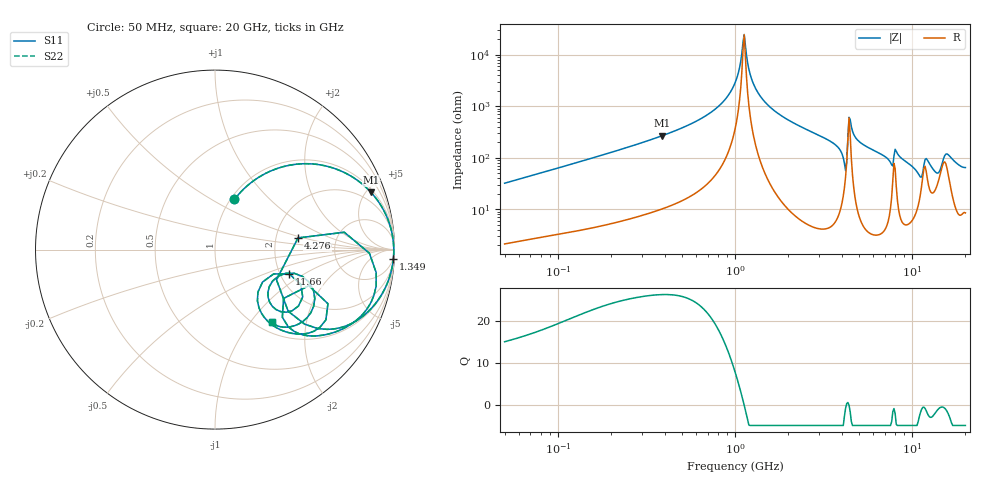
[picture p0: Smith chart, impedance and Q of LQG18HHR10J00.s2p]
!Murata Part Number: LQG18HHR10J00
!These Parameters are Measured in Series Mode Connection
!  o--[Z]--o
!Port1  Port2
!  o-------o
!Freq. Start=50[MHz] Stop=20[GHz], 401[Steps]
# Hz S RI R 50
!Freq.(Hz) S11(Real) S11(Imag) S21(Real) S21(Imag) S12(Real) S12(Imag) S22(Real) S22(Imag)
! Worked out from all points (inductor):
!   401 points, 50 MHz to 20 GHz, reference 50 ohm
!   read as one part in series: L = 101 nH near 51.52 MHz
!   highest Q = 26.4 at 389.2 MHz (marker M1), where L = 110 nH
!   self-resonance near 1.111 GHz
!   S11 on the Smith chart (normalised r, x): 50 MHz: 1.04, +0.64; 1.349 GHz: 3, -36; 4.276 GHz: 2.67, +0.44; 11.66 GHz: 2.24, -0.75; 20 GHz: 1.17, -1.28
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5e7  0.1085 0.2796  0.8915 -0.2796  0.8915 -0.2796  0.1085 0.2796
1.364002e8  0.4293 0.4725  0.5707 -0.4725  0.5707 -0.4725  0.4293 0.4725
3.721004e8  0.8573 0.3313  0.1427 -0.3313  0.1427 -0.3313  0.8573 0.3313
3.892024e8  0.8698 0.3182  0.1302 -0.3182  0.1302 -0.3182  0.8698 0.3182
7.411344e8  0.9783 0.1232  0.0217 -0.1232  0.0217 -0.1232  0.9783 0.1232
1e9  0.9944 0.0346  0.00562 -0.0346  0.00562 -0.0346  0.9944 0.0346
1.127304e9  0.996 -0.000643  0.00397 0.000643  0.00397 0.000643  0.996 -0.000643
1.23331e9  0.9955 -0.0273  0.00445 0.0273  0.00445 0.0273  0.9955 -0.0273
1.349283e9  0.9935 -0.0541  0.00646 0.0541  0.00646 0.0541  0.9935 -0.0541
2.728004e9  0.9048 -0.2863  0.0952 0.2863  0.0952 0.2863  0.9048 -0.2863
3.967106e9  0.626 -0.4445  0.374 0.4445  0.374 0.4445  0.626 -0.4445
4.275624e9  0.4626 0.065  0.5374 -0.065  0.5374 -0.065  0.4626 0.065
4.472136e9  0.8982 -0.1288  0.1018 0.1288  0.1018 0.1288  0.8982 -0.1288
4.608136e9  0.8855 -0.2552  0.1145 0.2552  0.1145 0.2552  0.8855 -0.2552
5.117541e9  0.7864 -0.3947  0.2136 0.3947  0.2136 0.3947  0.7864 -0.3947
7.442007e9  0.441 -0.4557  0.559 0.4557  0.559 0.4557  0.441 -0.4557
8.264682e9  0.5832 -0.4347  0.4168 0.4347  0.4168 0.4347  0.5832 -0.4347
9.745021e9  0.3595 -0.4441  0.6405 0.4441  0.6405 0.4441  0.3595 -0.4441
1.166392e10  0.414 -0.1363  0.586 0.1363  0.586 0.1363  0.414 -0.1363
1.375312e10  0.295 -0.2375  0.705 0.2375  0.705 0.2375  0.295 -0.2375
1.573793e10  0.5559 -0.2736  0.4441 0.2736  0.4441 0.2736  0.5559 -0.2736
2e10  0.3165 -0.4034  0.6835 0.4034  0.6835 0.4034  0.3165 -0.4034
